| TEXAS INSTRUMENTS INCORPORATED
| Standard Linear and Logic Group
| IBIS Model of SN74LVC139A
| DUAL 2-LINE TO 4-LINE DECODER/DEMULTIPLEXER
| This file contains package information for the following:
|  SOIC 16-pin (D) package as [Component] LVC139A_D
|  SSOP 16-pin (DB) package as [Component] LVC139A_DB
|  TVSOP 16-pin (DGV) package as [Component] LVC139A_DGV
|  SOP 16-pin (NS) package as [Component] LVC139A_NS
|  TSSOP 16-pin (PW) package as [Component] LVC139A_PW
|  VFBGA 20-pin (GQN) package as [Component] LVC139A_GQN
| This device can be powered at the following Vccs:
|  1.8 volt Vcc
|  2.5 volt Vcc
|  3.3 volt Vcc
| This file provides unique models under the [Model Selector] for each Vcc.
| For operation at a specific Vcc, select the appropriate model after each
| [Model Selector] keyword.
[IBIS Ver]   3.2
[Comment char]  |_char
[File Name]   sn74lvc139a.ibs
[File Rev]   1.1 | b_die
[Date]   July 31, 2002
[Source]   Data created from TI-SPICE simulations at TI-SLL.
[Notes]   The following is an IBIS list for the LVC139A_DL.
   Please contact sllibis@ti.com with questions and
   comments concerning SLL IBIS models.
[Disclaimer] Property of Texas Instruments Incorporated.  Unauthorized
   reproduction and/or distribution is strictly prohibited.
   This product is protected under copyright law.
   Created  2002, (C) Copyright  2002, Texas Instruments
   Incorporated, All Rights Reserved
   UNLESS THERE IS A SIGNED, WRITTEN AGREEMENT TO THE
   CONTRARY, TEXAS INSTRUMENTS (TI) IS PROVIDING THE IBIS
   MODELS  AND WITHOUT ANY WARRANTY, EXPRESSED OR
   IMPLIED.  TI assumes no liability for:
   1) the accuracy of the IBIS models provided to your
   company;
   2) the proper functioning of these IBIS Models in your
   design or for any resulting applications; or
   3) infringement of patents, copyrights or intellectual
   property rights resulting from your use of these IBIS
   models.
   TI provides IBIS Models as a service to our customers.
   You and your company shall not distribute, sell or give
   these models to anyone else without prior written
   permission from TI.
   TI reserves the right to make changes to our products or
   to discontinue any semiconductor product or service
   without notice, and advises our customers to obtain the
   latest version of relevant information to verify, before
   placing orders, that the information being relied on is
   current.
   Please be aware that your receipt and use of the IBIS
   information provided shall serve as acceptance of these
   terms and conditions.  If you do not accept these terms,
   you should return or destroy the IBIS models and any
   other accompanying information immediately.
| Component LVC139A_D 16-pin SOIC
[Component]   LVC139A_D
[Manufacturer]   Texas Instruments, Inc.
[Package]
|   typ   min   max
R_pkg   3.900e-02   2.800e-02   4.900e-02
L_pkg   3.453e-09   2.350e-09   4.375e-09
C_pkg   5.210e-13   2.540e-13   7.080e-13
[Pin]   signal_name   model_name   R_pin   L_pin   C_pin
1   1NG   LVC139A_OE   4.200e-02   4.336e-09   7.030e-13
2   1A   LVC139A_IN   4.900e-02   3.778e-09   6.340e-13
3   1B   LVC139A_IN   2.800e-02   3.449e-09   5.180e-13
4   1Y0   LVC139A_OUT   2.900e-02   2.393e-09   2.540e-13
5   1Y1   LVC139A_OUT   2.800e-02   2.350e-09   2.640e-13
6   1Y2   LVC139A_OUT   4.800e-02   3.312e-09   4.830e-13
7   1Y3   LVC139A_OUT   4.300e-02   3.629e-09   6.040e-13
8   GND   GND   4.400e-02   4.375e-09   7.080e-13
9   2Y3   LVC139A_OUT   4.200e-02   4.336e-09   7.030e-13
10   2Y2   LVC139A_OUT   4.900e-02   3.778e-09   6.340e-13
11   2Y1   LVC139A_OUT   2.800e-02   3.449e-09   5.180e-13
12   2Y0   LVC139A_OUT   2.900e-02   2.393e-09   2.550e-13
13   2B   LVC139A_IN   2.800e-02   2.350e-09   2.640e-13
14   2A   LVC139A_IN   4.800e-02   3.312e-09   4.830e-13
15   2NG   LVC139A_OE   4.300e-02   3.629e-09   6.040e-13
16   VCC   POWER   4.400e-02   4.375e-09   7.080e-13
| Component LVC139A_DB 16-pin SSOP
[Component]   LVC139A_DB
[Manufacturer]   Texas Instruments, Inc.
[Package]
|   typ   min   max
R_pkg   4.800e-02   4.600e-02   5.000e-02
L_pkg   3.536e-09   3.213e-09   3.798e-09
C_pkg   3.760e-13   3.140e-13   4.400e-13
[Pin]   signal_name   model_name   R_pin   L_pin   C_pin
1   1NG   LVC139A_OE   4.800e-02   3.797e-09   3.770e-13
2   1A   LVC139A_IN   4.600e-02   3.723e-09   4.400e-13
3   1B   LVC139A_IN   4.800e-02   3.409e-09   3.720e-13
4   1Y0   LVC139A_OUT   4.900e-02   3.213e-09   3.140e-13
5   1Y1   LVC139A_OUT   4.900e-02   3.213e-09   3.140e-13
6   1Y2   LVC139A_OUT   4.800e-02   3.409e-09   3.720e-13
7   1Y3   LVC139A_OUT   4.600e-02   3.723e-09   4.400e-13
8   GND   GND   4.800e-02   3.798e-09   3.770e-13
9   2Y3   LVC139A_OUT   4.800e-02   3.797e-09   3.770e-13
10   2Y2   LVC139A_OUT   4.600e-02   3.725e-09   4.400e-13
11   2Y1   LVC139A_OUT   4.800e-02   3.409e-09   3.720e-13
12   2Y0   LVC139A_OUT   4.900e-02   3.214e-09   3.140e-13
13   2B   LVC139A_IN   5.000e-02   3.216e-09   3.140e-13
14   2A   LVC139A_IN   4.800e-02   3.409e-09   3.720e-13
15   2NG   LVC139A_OE   4.700e-02   3.729e-09   4.400e-13
16   VCC   POWER   4.800e-02   3.797e-09   3.770e-13
| Component LVC139A_DGV 16-pin TVSOP
[Component]   LVC139A_DGV
[Manufacturer]   Texas Instruments, Inc.
[Package]
|   typ   min   max
R_pkg   3.900e-02   3.300e-02   4.500e-02
L_pkg   2.543e-09   2.320e-09   2.938e-09
C_pkg   3.860e-13   3.340e-13   4.490e-13
[Pin]   signal_name   model_name   R_pin   L_pin   C_pin
1   1NG   LVC139A_OE   3.500e-02   2.907e-09   4.170e-13
2   1A   LVC139A_IN   4.200e-02   2.558e-09   4.460e-13
3   1B   LVC139A_IN   3.800e-02   2.341e-09   3.450e-13
4   1Y0   LVC139A_OUT   3.800e-02   2.320e-09   3.340e-13
5   1Y1   LVC139A_OUT   3.900e-02   2.322e-09   3.340e-13
6   1Y2   LVC139A_OUT   3.800e-02   2.353e-09   3.420e-13
7   1Y3   LVC139A_OUT   4.000e-02   2.536e-09   4.410e-13
8   GND   GND   3.300e-02   2.897e-09   4.180e-13
9   2Y3   LVC139A_OUT   3.500e-02   2.927e-09   4.190e-13
10   2Y2   LVC139A_OUT   4.500e-02   2.632e-09   4.490e-13
11   2Y1   LVC139A_OUT   3.900e-02   2.368e-09   3.470e-13
12   2Y0   LVC139A_OUT   3.900e-02   2.330e-09   3.350e-13
13   2B   LVC139A_IN   3.900e-02   2.320e-09   3.350e-13
14   2A   LVC139A_IN   3.900e-02   2.361e-09   3.450e-13
15   2NG   LVC139A_OE   4.100e-02   2.573e-09   4.460e-13
16   VCC   POWER   3.500e-02   2.938e-09   4.200e-13
| Component LVC139A_NS 16-pin SOP
[Component]   LVC139A_NS
[Manufacturer]   Texas Instruments, Inc.
[Package]
|   typ   min   max
R_pkg   4.200e-02   3.500e-02   4.900e-02
L_pkg   3.147e-09   2.164e-09   4.219e-09
C_pkg   4.040e-13   2.410e-13   5.620e-13
[Pin]   signal_name   model_name   R_pin   L_pin   C_pin
1   1NG   LVC139A_OE   4.900e-02   4.215e-09   5.620e-13
2   1A   LVC139A_IN   4.600e-02   3.675e-09   4.800e-13
3   1B   LVC139A_IN   3.700e-02   2.527e-09   3.320e-13
4   1Y0   LVC139A_OUT   3.500e-02   2.164e-09   2.410e-13
5   1Y1   LVC139A_OUT   3.500e-02   2.164e-09   2.410e-13
6   1Y2   LVC139A_OUT   3.700e-02   2.527e-09   3.320e-13
7   1Y3   LVC139A_OUT   4.600e-02   3.675e-09   4.800e-13
8   GND   GND   4.900e-02   4.215e-09   5.620e-13
9   2Y3   LVC139A_OUT   4.900e-02   4.219e-09   5.620e-13
10   2Y2   LVC139A_OUT   4.600e-02   3.679e-09   4.800e-13
11   2Y1   LVC139A_OUT   3.700e-02   2.531e-09   3.330e-13
12   2Y0   LVC139A_OUT   3.500e-02   2.168e-09   2.410e-13
13   2B   LVC139A_IN   3.500e-02   2.168e-09   2.410e-13
14   2A   LVC139A_IN   3.700e-02   2.531e-09   3.330e-13
15   2NG   LVC139A_OE   4.600e-02   3.679e-09   4.800e-13
16   VCC   POWER   4.900e-02   4.219e-09   5.620e-13
| Component LVC139A_PW 16-pin TSSOP
[Component]   LVC139A_PW
[Manufacturer]   Texas Instruments, Inc.
[Package]
|   typ   min   max
R_pkg   4.500e-02   3.800e-02   5.100e-02
L_pkg   2.593e-09   2.447e-09   3.080e-09
C_pkg   2.810e-13   2.430e-13   3.770e-13
[Pin]   signal_name   model_name   R_pin   L_pin   C_pin
1   1NG   LVC139A_OE   4.000e-02   3.080e-09   3.770e-13
2   1A   LVC139A_IN   3.800e-02   2.458e-09   2.810e-13
3   1B   LVC139A_IN   5.100e-02   2.512e-09   2.550e-13
4   1Y0   LVC139A_OUT   5.100e-02   2.447e-09   2.430e-13
5   1Y1   LVC139A_OUT   5.100e-02   2.447e-09   2.430e-13
6   1Y2   LVC139A_OUT   5.100e-02   2.512e-09   2.550e-13
7   1Y3   LVC139A_OUT   3.800e-02   2.458e-09   2.810e-13
8   GND   GND   4.000e-02   3.080e-09   3.770e-13
9   2Y3   LVC139A_OUT   3.900e-02   2.832e-09   3.160e-13
10   2Y2   LVC139A_OUT   3.800e-02   2.460e-09   2.790e-13
11   2Y1   LVC139A_OUT   5.100e-02   2.512e-09   2.550e-13
12   2Y0   LVC139A_OUT   5.100e-02   2.447e-09   2.430e-13
13   2B   LVC139A_IN   5.100e-02   2.447e-09   2.430e-13
14   2A   LVC139A_IN   5.100e-02   2.512e-09   2.550e-13
15   2NG   LVC139A_OE   3.800e-02   2.459e-09   2.790e-13
16   VCC   POWER   3.900e-02   2.832e-09   3.160e-13
| Component LVC139A_GQN 20-pin VFBGA
[Component]   LVT139A_GQN
[Manufacturer] Texas Instruments, Inc.
[Package]
|   typ   min   max
R_pkg   4.300e-02   3.300e-02   6.100e-02
L_pkg   1.317e-09   8.960e-10   2.088e-09
C_pkg   1.130e-13   6.400e-14   1.900e-13
[Pin]   signal_name   model_name   R_pin   L_pin   C_pin
A2   1NG   LVC139A_OE   3.800e-02   1.199e-09   1.210e-13
A1   1A   LVC139A_IN   4.000e-02   1.067e-09   1.020e-13
B3   NC   NC   6.100e-02   1.999e-09   1.900e-13
B1   1B   LVC139A_IN   3.300e-02   9.630e-10   7.100e-14
C2   1Y0   LVC139A_OUT   4.900e-02   1.523e-09   1.230e-13
C1   1Y1   LVC139A_OUT   3.300e-02   8.960e-10   6.400e-14
D3   NC   NC   6.100e-02   1.899e-09   1.640e-13
D1   1Y2   LVC139A_OUT   3.300e-02   8.980e-10   6.700e-14
E2   1Y3   LVC139A_OUT   4.900e-02   1.514e-09   1.280e-13
E1   GND   GND   3.600e-02   1.006e-09   9.400e-14
E3   2Y3   LVC139A_OUT   4.900e-02   1.683e-09   1.460e-13
E4   2Y2   LVC139A_OUT   3.300e-02   1.121e-09   8.900e-14
D2   NC   NC   6.100e-02   2.088e-09   1.730e-13
D4   2Y1   LVC139A_OUT   3.300e-02   1.027e-09   7.100e-14
C3   2Y0   LVC139A_OUT   4.900e-02   1.558e-09   1.240e-13
C4   2B   LVC139A_IN   3.300e-02   9.280e-10   6.700e-14
B2   NC   NC   6.100e-02   1.921e-09   1.770e-13
B4   2A   LVC139A_IN   3.300e-02   9.010e-10   7.700e-14
A4   2NG   LVC139A_OE   3.700e-02   9.900e-10   9.800e-14
A3   VCC   POWER   3.500e-02   1.168e-09   1.190e-13
| Model LVC139A_IN
[Model Selector]   LVC139A_IN
LVC139A_IN_18   1.8 volt Vcc
LVC139A_IN_25   2.5 volt Vcc
LVC139A_IN_33   3.3 volt Vcc
| Model LVC139A_OE
[Model Selector]   LVC139A_OE
LVC139A_OE_18   1.8 volt Vcc
LVC139A_OE_25   2.5 volt Vcc
LVC139A_OE_33   3.3 volt Vcc
| Model LVC139A_OUT
[Model Selector]   LVC139A_OUT
LVC139A_OUT_18   1.8 volt Vcc
LVC139A_OUT_25   2.5 volt Vcc
LVC139A_OUT_33   3.3 volt Vcc
| Models and submodels in the file (9): LVC139A_IN_18 (Input), LVC139A_IN_25 (Input), LVC139A_IN_33 (Input), LVC139A_OE_18 (Input), LVC139A_OE_25 (Input), LVC139A_OE_33 (Input), LVC139A_OUT_18 (Output), LVC139A_OUT_25 (Output), LVC139A_OUT_33 (Output)
